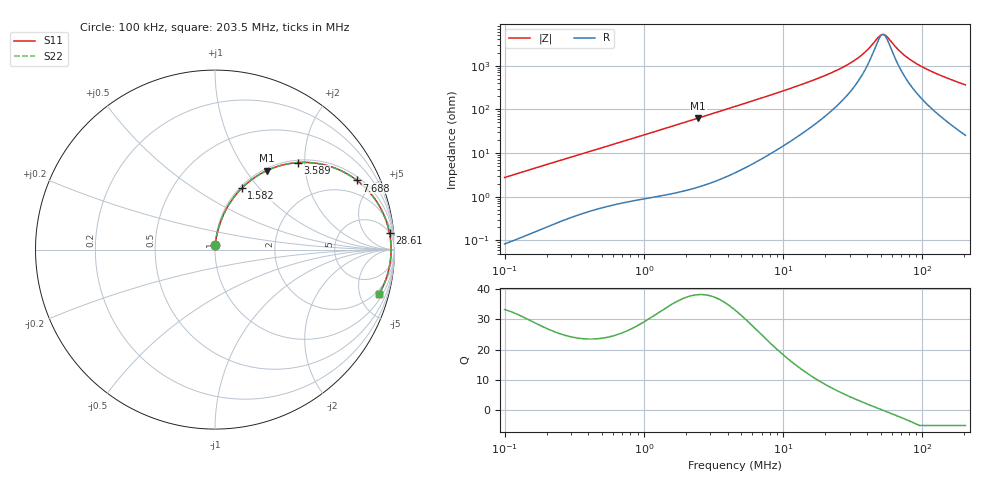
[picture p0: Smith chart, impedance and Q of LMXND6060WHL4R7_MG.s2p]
! LMXND6060WHL4R7_MG  S-PARAMETER MODEL  ( General Type )
! Model Generated by TAIYO YUDEN Corporation (http://www.ty-top.com)
! Version 1.0
! TAIYO YUDEN Control No. 191025NI43SB-FBB
! Copyright(c) 2019 TAIYO YUDEN CO.,LTD. All Rights Reserved.
! Product Description (link to TY-COMPAS)
! https://ds.yuden.co.jp/TYCOMPAS/or/detail?pn=LMXND6060WHL4R7MMG&u=M
! Products Name : Inductors
! Characteristics :
!  Inductance : 4.7 uH , SRF(min) : 39 MHz , DC Resistance(max) : 0.0403 Ohm
!  Rated Current : Saturation :2700 mA , Temp Rise : 3000 mA
!  Case Size : 6.0 x 6.0 / 0.236 x 0.236 [mm/inch] , Thickness : 2.8 / 0.11 [mm/inch]
!  (Conditions: Temperature = 25 degC , DC Bias Current/Voltage = 0A / 0V)
! External Node Assignments :
!  1  o---GGG---o  2
! GND o---------o GND
! Frequency Range : 0.1MHz  -  203.457813MHz  [ 402 STEP ]
# MHz S RI R 50
! Freq[MHz].  S11 Real  S11 Imag  S21 Real  S21 Imag  S12 Real  S12 Imag  S22 Real  S22 Imag
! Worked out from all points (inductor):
!   401 points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, 100 kHz to 203.5 MHz, reference 50 ohm
!   read as one part in series: L = 4.36 uH near 103.9 kHz
!   highest Q = 38.1 at 2.452 MHz (marker M1), where L = 4.08 uH
!   self-resonance near 52.05 MHz
!   S11 on the Smith chart (normalised r, x): 100 kHz: 1.00, +0.06; 1.582 MHz: 1.02, +0.81; 3.589 MHz: 1.05, +1.84; 7.688 MHz: 1.17, +4.01; 28.61 MHz: 5, +20; 203.5 MHz: 1.51, -7.24
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0.1  0.00158 0.0274  0.9984 -0.0274  0.9984 -0.0274  0.00158 0.0274
0.358236  0.013 0.094  0.987 -0.094  0.987 -0.094  0.013 0.094
0.697688  0.0385 0.1739  0.9615 -0.1739  0.9615 -0.1739  0.0385 0.1739
1.283332  0.1059 0.2926  0.8941 -0.2926  0.8941 -0.2926  0.1059 0.2926
1.582421  0.1491 0.3421  0.8509 -0.3421  0.8509 -0.3421  0.1491 0.3421
2.452219  0.2887 0.4402  0.7113 -0.4402  0.7113 -0.4402  0.2887 0.4402
3.589078  0.4606 0.4848  0.5394 -0.4848  0.5394 -0.4848  0.4606 0.4848
4.51063  0.5721 0.4799  0.4279 -0.4799  0.4279 -0.4799  0.5721 0.4799
7.688301  0.7909 0.3855  0.2091 -0.3855  0.2091 -0.3855  0.7909 0.3855
10.83208  0.8791 0.2978  0.1209 -0.2978  0.1209 -0.2978  0.8791 0.2978
16.15871  0.9374 0.2012  0.0626 -0.2012  0.0626 -0.2012  0.9374 0.2012
22.33659  0.9619 0.1349  0.0381 -0.1349  0.0381 -0.1349  0.9619 0.1349
28.61161  0.9724 0.0911  0.0276 -0.0911  0.0276 -0.0911  0.9724 0.0911
38.07238  0.9789 0.0459  0.0211 -0.0459  0.0211 -0.0459  0.9789 0.0459
49.70575  0.981 0.00667  0.019 -0.00667  0.019 -0.00667  0.981 0.00667
51.63557  0.9811 0.00116  0.0189 -0.00116  0.0189 -0.00116  0.9811 0.00116
53.64032  0.9811 -0.00436  0.0189 0.00436  0.0189 0.00436  0.9811 -0.00436
57.88634  0.9809 -0.0154  0.0191 0.0154  0.0191 0.0154  0.9809 -0.0154
71.37714  0.9789 -0.0464  0.0211 0.0464  0.0211 0.0464  0.9789 -0.0464
91.42912  0.9736 -0.0853  0.0264 0.0853  0.0264 0.0853  0.9736 -0.0853
131.2916  0.9575 -0.1502  0.0425 0.1502  0.0425 0.1502  0.9575 -0.1502
203.4578  0.9146 -0.2466  0.0854 0.2466  0.0854 0.2466  0.9146 -0.2466
